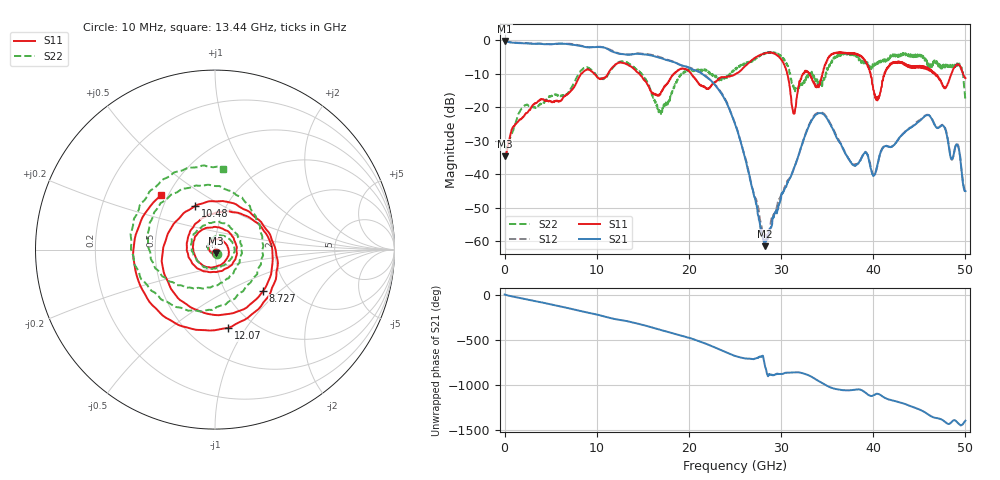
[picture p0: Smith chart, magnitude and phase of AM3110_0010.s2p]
# Hz S DB R 50.0
!freq dBS11 angS11 dBS21 angS21 dBS12 angS12 dBS22 angS22
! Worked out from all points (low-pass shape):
!   1601 points, 10 MHz to 50 GHz, reference 50 ohm
!   highest |S21| = -0.18 dB at 10 MHz (marker M1); lowest = -61.5 dB at 28.25 GHz (marker M2)
!   |S21| within 3 dB of the highest: start of sweep to 11.55 GHz
!   lowest |S11| = -34.6 dB at 10 MHz (marker M3), VSWR 1.04, Z = 50.4 - j1.83 ohm
!   |S11| at or under -10 dB: start of sweep to 8.316 GHz; 14.6 GHz to 18.38 GHz (3.782 GHz wide, 22.9 % of centre); 20.27 GHz to 25.1 GHz (4.83 GHz wide, 21.3 % of centre)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
!   |S22| runs from -32.3 to -3.5 dB; largest |S21 - S12| = 0.025
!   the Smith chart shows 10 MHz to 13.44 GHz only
!   S11 on the Smith chart (normalised r, x): 10 MHz: 1.01, -0.04; 8.727 GHz: 1.48, -0.78; 10.48 GHz: 0.72, +0.38; 12.07 GHz: 0.77, -0.83; 13.44 GHz: 0.46, +0.34
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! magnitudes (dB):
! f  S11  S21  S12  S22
! 10 MHz  -34.6  -0.2  0.0  -31.0
! 1.978 GHz  -22.9  -0.9  -0.8  -20.0
! 8.352 GHz  -9.9  -1.7  -1.6  -8.8
! 8.727 GHz  -9.0  -2.0  -1.9  -8.1
! 10.48 GHz  -11.4  -2.0  -1.9  -11.5
! 12.07 GHz  -7.1  -3.7  -3.5  -7.1
! 13.44 GHz  -7.4  -4.3  -4.2  -6.9
! 16.69 GHz  -16.4  -5.1  -4.8  -20.2
! 19.57 GHz  -8.6  -7.7  -7.7  -9.2
! 25 GHz  -10.2  -25.0  -24.8  -8.7
! 28.25 GHz  -3.9  -61.5  -57.9  -4.0
! 30.25 GHz  -6.7  -45.3  -45.1  -5.3
! 31.38 GHz  -21.8  -38.3  -38.4  -14.1
! 32.38 GHz  -9.9  -30.2  -30.2  -12.3
! 33.35 GHz  -11.3  -23.8  -23.5  -9.4
! 37.88 GHz  -3.8  -37.3  -37.3  -4.1
! 40.03 GHz  -14.8  -40.5  -40.1  -7.7
! 41.69 GHz  -7.7  -31.8  -31.7  -5.8
! 46.03 GHz  -8.7  -22.3  -22.3  -6.9
! 47.78 GHz  -14.4  -26.3  -26.0  -7.7
! 49.16 GHz  -7.2  -31.3  -31.1  -7.5
! 50 GHz  -11.3  -45.0  -45.4  -17.9
